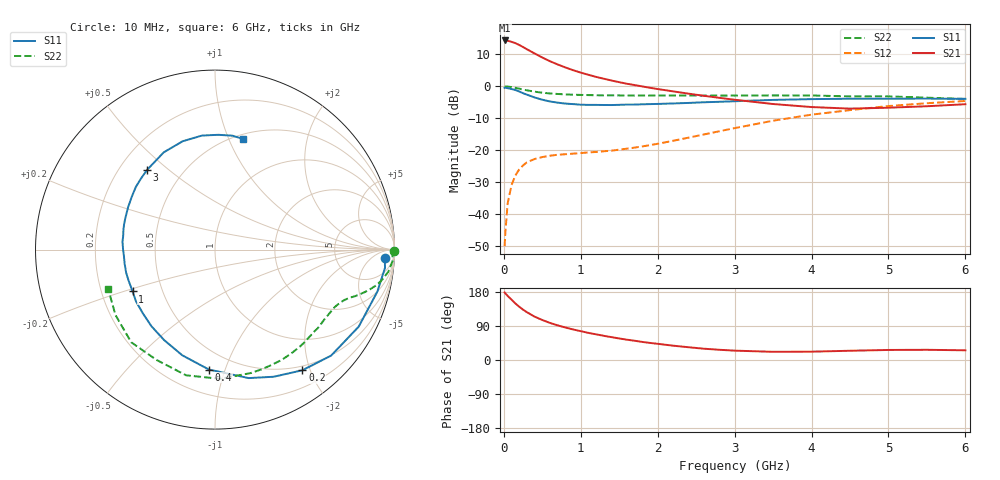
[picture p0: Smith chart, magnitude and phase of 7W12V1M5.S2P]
! Infineon Technologies  Discrete & RF Semiconductors
! BFS17W
! Si NPN RF Bipolar Junction Transistor in SOT323
! VCE = 12 V  IC = 1.5 mA
! Common Emitter S-Parameters:  August  1999
# GHz  S  MA  R  50
!  f  S11  S21  S12  S22
! GHz  MAG  ANG  MAG  ANG  MAG  ANG  MAG  ANG
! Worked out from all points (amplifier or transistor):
!   36 points, 10 MHz to 6 GHz, reference 50 ohm
!   highest |S21| = 14.4 dB at 10 MHz (marker M1)
!   |S21| within 3 dB of that: start of sweep to 317.9 MHz
!   unconditionally stable (mu >= 1): 952.6 MHz to 2.718 GHz; 4.415 GHz to end of sweep
!   at 250 MHz: K = 0.30, MSG = 18.6 dB, |S12| = -24.8 dB
!   at 1.4 GHz: K = 1.24, MAG = 8.0 dB, |S12| = -20.2 dB
!   at 6 GHz: K = 1.07, MAG = -2.2 dB, |S12| = -4.6 dB
!   S11 on the Smith chart (normalised r, x): 10 MHz: 20, -18; 200 MHz: 0.43, -1.88; 400 MHz: 0.36, -0.88; 1 GHz: 0.34, -0.21; 3 GHz: 0.31, +0.42; 6 GHz: 0.55, +1.13
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0.01  0.9464 -2.8  5.25 178.4  0.0031 82.3  0.9999 -0.3
0.02  0.9528 -6.1  5.225 175.7  0.0052 88.4  0.9895 -1.5
0.05  0.9344 -14.5  5.201 169.1  0.0146 81.6  0.9913 -3.7
0.1  0.9085 -28.2  4.988 159.2  0.0282 75.3  0.9741 -7.2
0.15  0.876 -42.4  4.762 149.2  0.0399 67.3  0.9469 -10.2
0.2  0.83 -54.1  4.456 140.6  0.0497 62.0  0.9199 -12.5
0.25  0.7803 -65.2  4.138 132.9  0.0574 56.2  0.8912 -14.4
0.3  0.7401 -75.3  3.819 126.1  0.0642 52.9  0.8665 -15.9
0.4  0.6691 -92.9  3.282 114.4  0.0724 46.7  0.8243 -18.3
0.5  0.6165 -107.2  2.833 105.5  0.0776 43.3  0.7945 -19.8
0.6  0.5785 -119.3  2.476 97.8  0.0815 41.2  0.7735 -21.3
0.7  0.5545 -129.8  2.204 91.4  0.0844 41.3  0.759 -22.8
0.8  0.5362 -138.6  1.98 85.7  0.086 41.3  0.747 -24.4
1  0.5151 -153.1  1.642 76.1  0.0897 42.8  0.7338 -27.6
1.1  0.5115 -160.2  1.517 71.5  0.0919 44.4  0.7288 -29.6
1.6  0.5172 175.1  1.098 53.6  0.1051 54.6  0.7167 -39.7
2.2  0.5387 154.0  0.834 37.8  0.1398 67.5  0.7179 -53.6
3  0.5837 130.3  0.616 24.7  0.2209 73.2  0.716 -73.8
3.5  0.6126 117.8  0.528 21.6  0.2886 71.1  0.7207 -87.6
4.5  0.6395 96.5  0.447 24.4  0.4234 59.4  0.6957 -117.8
5.5  0.6419 81.3  0.487 26.9  0.5432 45.3  0.6636 -146.7
6  0.6361 75.7  0.524 25.6  0.5894 38.5  0.6342 -159.7
